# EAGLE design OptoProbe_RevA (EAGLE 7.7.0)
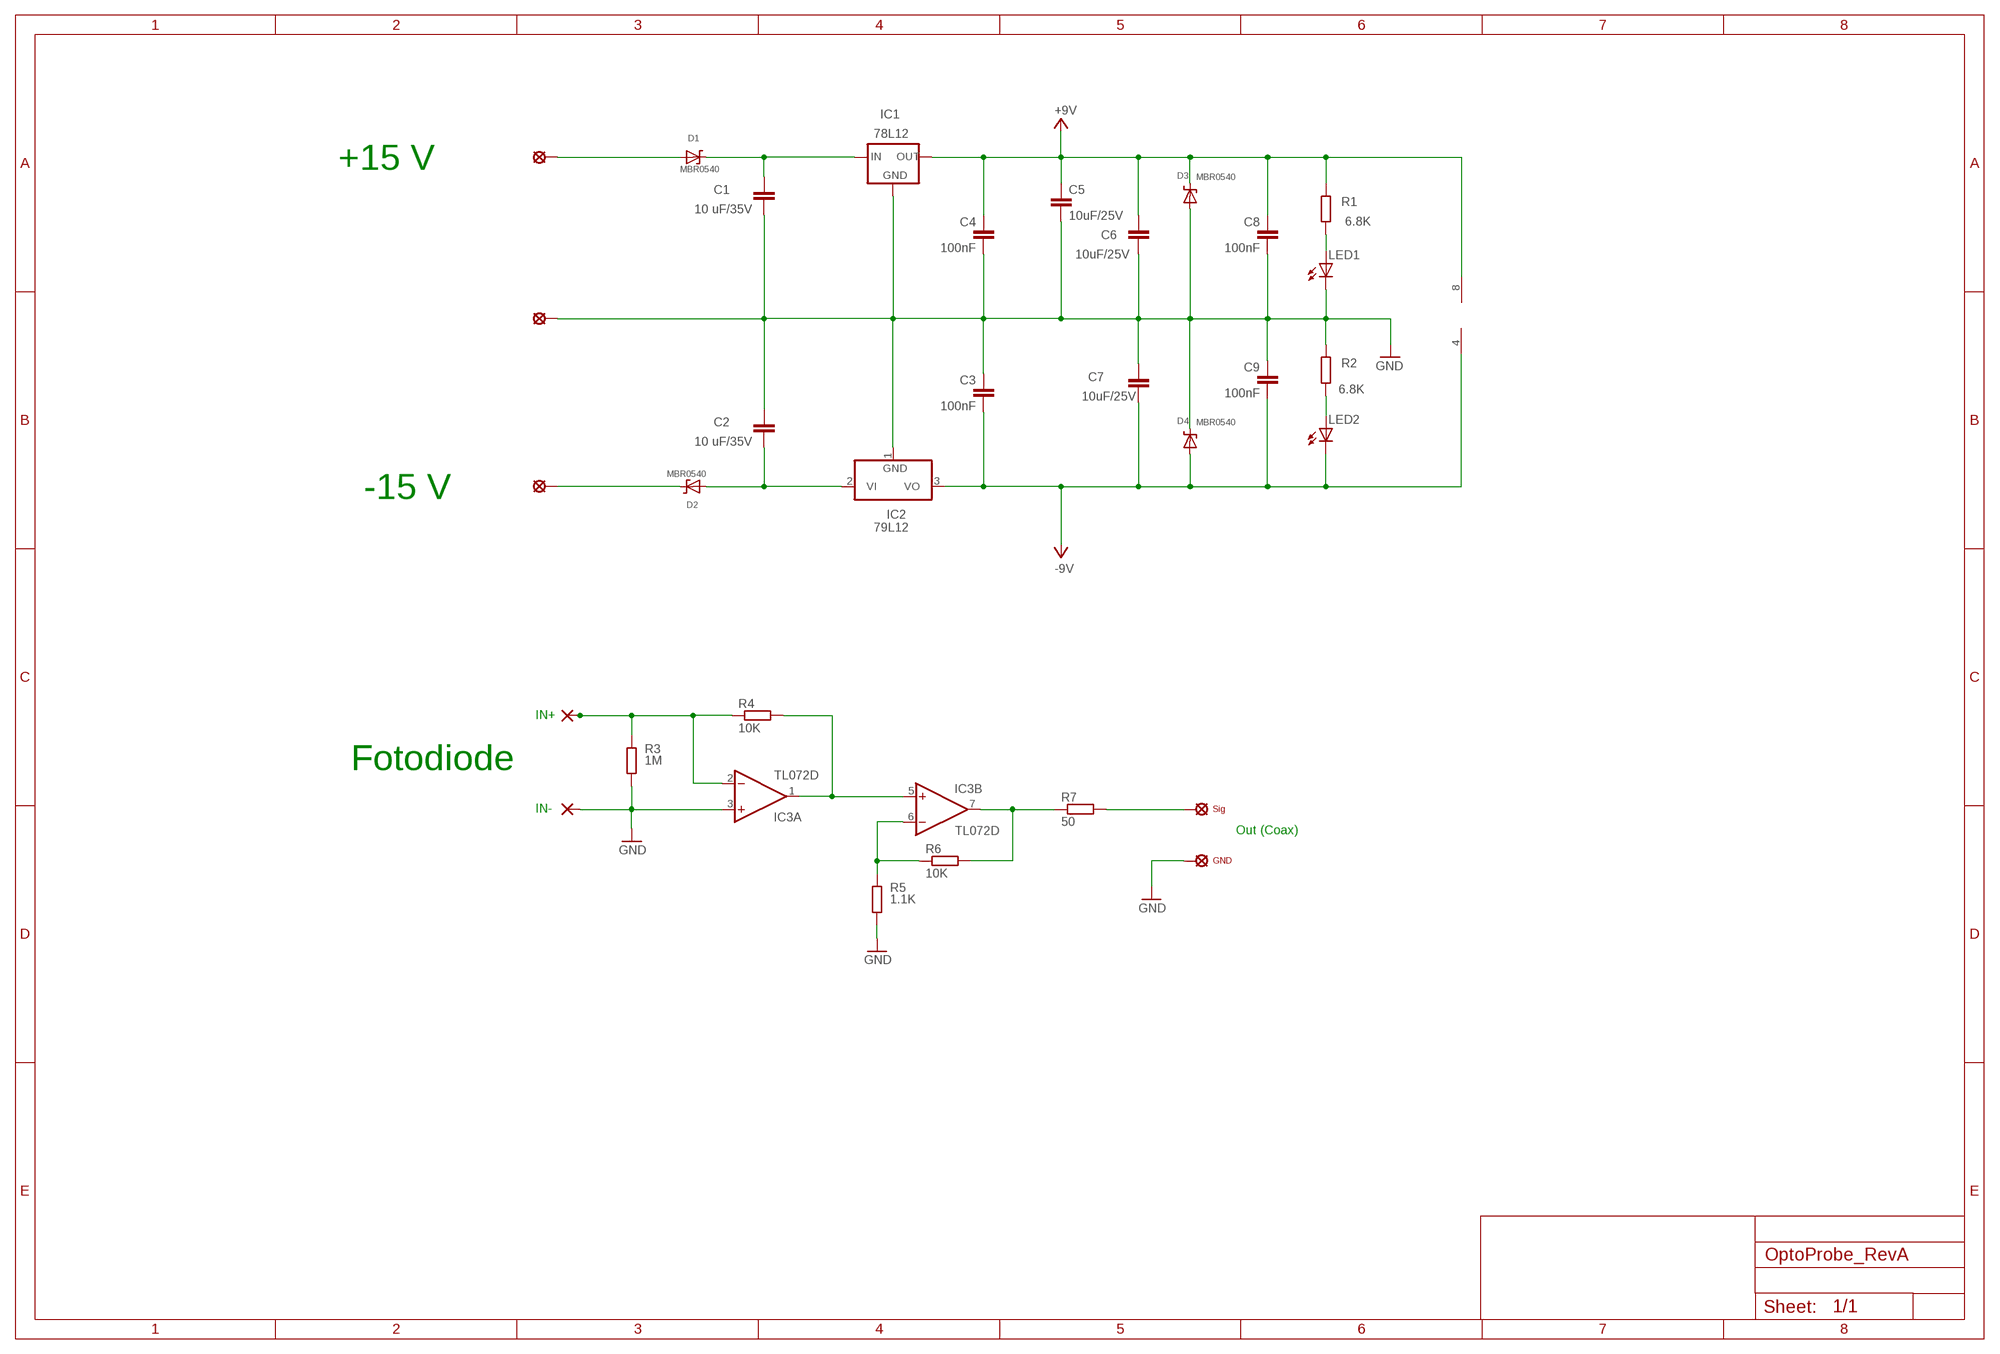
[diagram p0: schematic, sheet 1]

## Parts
+5VIN  SE2.5_1.0  [SE2.5_1.0]
C1  10 uF/35V  C-EUC1206  [C1206]
C2  10 uF/35V  C-EUC1206  [C1206]
C3  100nF  C-EUC0603  [C0603]
C4  100nF  C-EUC0603  [C0603]
C5  10uF/25V  C-EUC0805  [C0805]
C6  10uF/25V  C-EUC0805  [C0805]
C7  10uF/25V  C-EUC0805  [C0805]
C8  100nF  C-EUC0603  [C0603]
C9  100nF  C-EUC0603  [C0603]
D1  MBR0540  D-SCHTTKY_PMEG2005EH_SOD-123  [SOD-123]
D2  MBR0540  D-SCHTTKY_PMEG2005EH_SOD-123  [SOD-123]
D3  MBR0540  D-SCHTTKY_PMEG2005EH_SOD-123  [SOD-123]
D4  MBR0540  D-SCHTTKY_PMEG2005EH_SOD-123  [SOD-123]
GND  SE2.5_1.0  [SE2.5_1.0]
GND3  SE2.5_1.0  [SE2.5_1.0]
IC1  78L12  78LXX  [78LXX]
IC2  79L12  79L05Z  [TO92]
IC3  TL072D  [SO08]
IN+  SMD3X2  [SMD3.00X2.00]
IN-  SMD3X2  [SMD3.00X2.00]
LED1  LEDCHIPLED_0603  [CHIPLED_0603]
LED2  LEDCHIPLED_0603  [CHIPLED_0603]
R1  6.8K  R-EU_R0603  [R0603]
R2  6.8K  R-EU_R0603  [R0603]
R3  1M  R-EU_R0603  [R0603]
R4  10K  R-EU_R0603  [R0603]
R5  1.1K  R-EU_R0603  [R0603]
R6  10K  R-EU_R0603  [R0603]
R7  50  R-EU_R0603  [R0603]
U$3  RG178BU  [RG178BU]

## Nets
+9V: C4.1 C5.1 C6.1 C8.1 D3.K IC1.OUT IC3.8(P:V+) R1.1
+11.5V: C1.1 D1.K IC1.IN
-9V: C3.2 C7.2 C9.2 D4.A IC2.3(VO) IC3.4(P:V-) LED2.C
GND: C1.2 C2.1 C3.1 C4.2 C5.2 C6.2 C7.1 C8.2 C9.1 D3.A D4.K GND.MP IC1.GND IC2.1(GND) IC3.3(A:+IN) IN-.1(P) LED1.C R2.1 R3.2 R5.2 U$3.P$3(GND) U$3.P$4(GND) U$3.P$5(GND) U$3.P$6(GND) U$3.P$7(GND) U$3.P$8(GND) U$3.P$9(GND) U$3.P$10(GND)
N$1: C2.2 D2.A IC2.2(VI)
N$2: LED2.A R2.2
N$3: D2.K GND3.MP
N$5: IC3.2(A:-IN) IN+.1(P) R3.1 R4.1
N$6: IC3.1(A:OUT) IC3.5(B:+IN) R4.2
N$7: IC3.6(B:-IN) R5.1 R6.1
N$8: IC3.7(B:OUT) R6.2 R7.1
N$16: LED1.A R1.2
N$29: +5VIN.MP D1.A
N$34: R7.2 U$3.P$1(SIG) U$3.P$2(SIG)

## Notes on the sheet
- +15 V
- -15 V
- Fotodiode
- Out (Coax)

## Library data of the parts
+5VIN GND GND3 = solpad2:SE2.5_1.0: SOLDER PAD
C1-C9 = rcl:C-EU: CAPACITOR, European symbol
D1-D4 = diodes:D-SCHTTKY_*_: Schottky diode; LOAD: 500mA; PARTNO: DIS-PMEG2005EH; RATE: 355mW; SIZE: (SOD-123); VAL: PMEG2005EH; VOLT: 20V
IC1 = v-reg:78LXX: VOLTAGE REGULATOR
IC2 = linear:79*: Negative VOLTAGE REGULATOR
IC3 = linear:TL072: OP AMP
IN+ IN- = wirepad2:SMD3X2: SMD PAD 3x2mm
LED1 LED2 = led2:LED: LED
R1-R7 = rcl:R-EU_: RESISTOR, European symbol
U$3 = solpad2:RG178BU: SMD-Pads für SMA-Koaxkabel RG178BU

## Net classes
3 gnd: clearance 0.12 mm to class 0, clearance 0.3 mm to class 1, clearance 0.1 mm to class 2

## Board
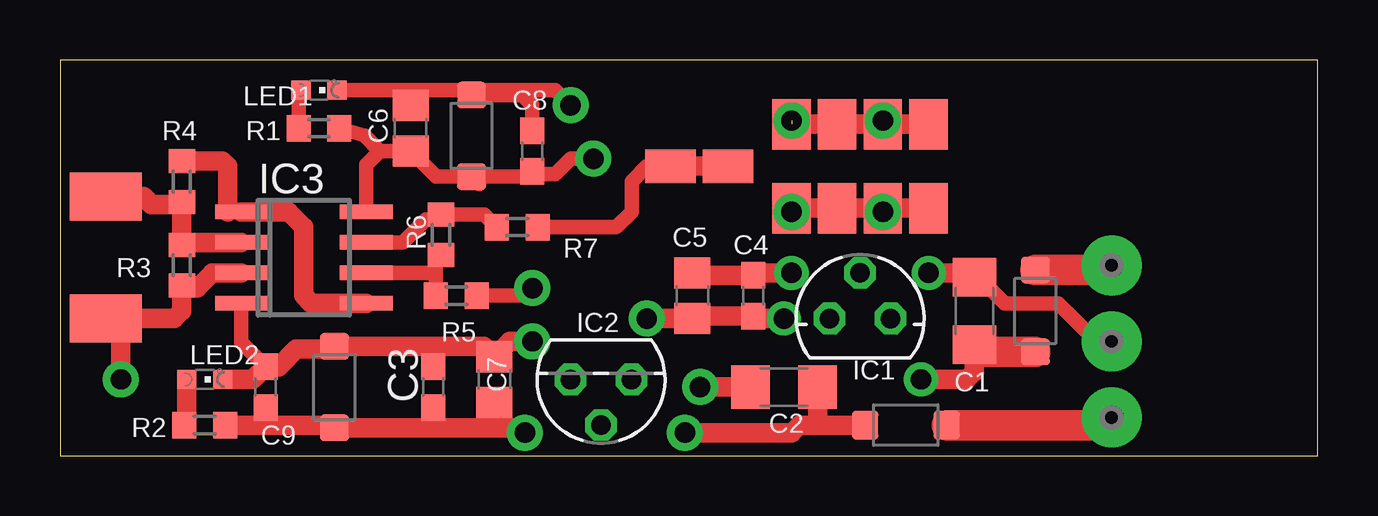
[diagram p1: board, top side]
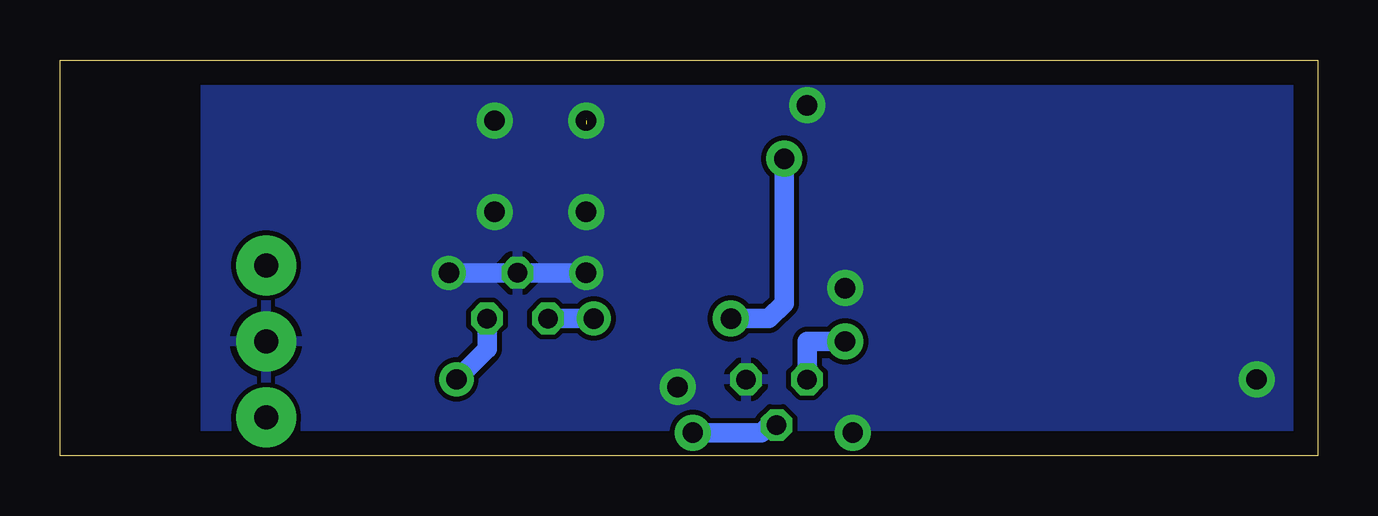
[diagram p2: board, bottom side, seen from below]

Size 52.4 x 16.5 mm. Coordinates in mm from the lower left corner, seen from the top.
Outline: 0,0 52.4,0 52.4,16.5 0,16.5 0,0
Copper layers (1*16): Top 0.035mm / dielectric 1.5mm / Bottom 0.035mm
Design rules "default": minimum track width 10mil, minimum drill 24mil, track to track 8mil, track to pad 8mil, pad to pad 8mil, via to via 8mil, smd to smd 8mil, copper to edge 40mil, drill to drill 8mil, minimum pad ring 10mil, minimum via ring 8mil, stop-mask expansion 4mil, vias tented up to drill 0mil, thermal gap 10mil

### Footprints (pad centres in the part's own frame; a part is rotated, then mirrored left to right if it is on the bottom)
SE2.5_1.0 = drill 1 pad 2.5: MP 0,0
C1206 = smd 1.6 x 1.8: 1 -1.4,0; 2 1.4,0
C0603 = smd 1.1 x 1: 1 -0.85,0; 2 0.85,0
C0805 = smd 1.3 x 1.5: 1 -0.95,0; 2 0.95,0
SOD-123 = smd 1.1 x 1.2: A 1.7,0; K -1.7,0
78LXX = drill 0.813 octagon: GND 0,1.905; IN 1.27,0; OUT -1.27,0
TO92 = drill 0.813 octagon: 1 -1.27,0; 2 0,1.905; 3 1.27,0
SO08 = smd 0.6 x 2.2: 1 -1.905,-2.6; 2 -0.635,-2.6; 3 0.635,-2.6; 4 1.905,-2.6; 5 1.905,2.6; 6 0.635,2.6; 7 -0.635,2.6; 8 -1.905,2.6
SMD3.00X2.00 = smd 2 x 3: 1 0,0
CHIPLED_0603 = smd 0.8 x 0.8: A 0,-0.75; C 0,0.75
R0603 = smd 1 x 1.1: 1 -0.85,0; 2 0.85,0
RG178BU = smd 1.4 x 2.1: P$1 0,6; P$2 0,3.6 | smd 2.1 x 1.6: P$3 -1.75,0.95; P$4 1.75,0.95; P$5 -1.75,-0.95; P$6 1.75,-0.95; P$7 -1.75,-2.85; P$8 1.75,-2.85; P$9 -1.75,-4.75; P$10 1.75,-4.75

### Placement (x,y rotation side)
+5VIN  43.81,7.94 0 top
C1  38.1,6.03 90 top
C2  30.16,2.86 0 top
C3  15.56,2.86 90 top
C4  28.89,6.67 90 top
C5  26.35,6.67 90 top
C6  14.61,13.65 90 top
C7  18.1,3.17 90 top
C8  19.69,12.7 90 top
C9  8.57,2.86 90 top
D1  40.64,6.03 90 top
D2  35.24,1.27 180 top
D3  17.14,13.34 90 top
D4  11.43,2.86 90 top
GND  43.81,4.76 0 top
GND3  43.81,1.59 0 top
IC1  33.34,5.71 0 top
IC2  22.54,3.17 180 top
IC3  10.16,8.26 270 top
IN+  1.91,10.79 90 top
IN-  1.91,5.71 90 top
LED1  10.8,15.24 270 top
LED2  6.03,3.17 270 top
R1  10.8,13.65 180 top
R2  6.03,1.27 180 top
R3  5.08,7.94 270 top
R4  5.08,11.43 90 top
R5  16.51,6.67 0 top
R6  15.88,9.21 90 top
R7  19.05,9.53 0 top
U$3  31.43,12.06 90 top

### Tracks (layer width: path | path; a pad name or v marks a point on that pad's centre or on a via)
+9V  (via drill 0.85 pad 1.42, 0.85 pad 1.5)
  Top 0.61: 17.46,11.32 D3.K | D3.K 19.47,11.63 C8.1 19.79,11.75 20.64,11.75 21.27,12.38 v22.22,12.38 | D3.K 15.67,11.63 C6.1 13.33,12.7 | 13.33,12.7 12.7,13.34 R1.1 | IC3.8 12.76,12.13 13.33,12.7
  Top 0.813: v24.45,5.71 v24.45,5.72 C5.1 26.45,5.82 C4.1 29,5.71 v30.16,5.71
  Bottom 0.813: v24.45,5.71 22.86,5.71 22.22,6.35 v22.22,12.38 | IC1.OUT v30.16,5.71
+11.5V  (via drill 0.85 pad 1.42)
  Top 0.813: v35.88,3.17 37.78,3.17 38.1,3.49 C1.1
  Top 1.27: D1.K 38.4,4.33 C1.1
  Bottom 0.813: IC1.IN 34.61,4.45 v35.88,3.17
-9V  (via drill 0.85 pad 1.5)
  Top 0.406: 14.27,4.56 14.23,4.6 | 17.67,4.56 C7.2
  Top 0.61: IC3.4 7.56,4.72 C9.2
  Top 0.813: D4.A 14.27,4.56 | D4.A 15.56,4.56 | 15.56,4.56 17.67,4.56 | LED2.C 8.04,3.17 C9.2 9.11,3.71 9.84,4.45 11.32,4.45 D4.A | v19.69,4.76 18.74,4.76 C7.2 | C3.2 15.56,4.56
  Bottom 0.813: IC2.3 21.27,4.76 v19.69,4.76
GND  (via drill 0.85 pad 1.42, 0.85 pad 1.5)  (1 unrouted)
  Top 0.406: 5.71,6.99 5.18,6.99 R3.2
  Top 0.61: 14.61,15.24 LED1.C 20.64,15.24 v21.27,14.61 | 14.61,15.24 16.94,15.24 D3.A 19.26,15.04 19.69,14.61 C8.2 | C6.2 14.61,15.24 | C1.2 38.29,7.43 39.37,6.35 41.59,6.35 43.18,4.76 GND.MP | R5.2 19.37,6.67 v19.69,6.99
  Top 0.813: U$3.P$4 U$3.P$6 U$3.P$8 U$3.P$10 | U$3.P$3 U$3.P$5 U$3.P$7 U$3.P$9 | C5.2 26.45,7.52 C4.2 29,7.62 v30.48,7.62 | C2.1 v26.67,2.86 | C1.2 38.1,7.62 v36.19,7.62 | IC3.3 6.35,7.62 5.71,6.99 | IN-.1 2.54,5.71 | R3.2 5.08,6.03 4.76,5.71 2.54,5.71 | R2.1 8.57,1.27 | 8.57,1.27 11.32,1.27 D4.K 15.56,1.16 | C9.1 8.57,1.27 | 15.56,1.16 18.1,1.16 | 18.1,1.16 19.16,1.16 v19.37,0.95 | C7.1 18.1,1.16 | C3.1 15.56,1.16 | 2.54,5.71 v2.54,3.17
  Top 1.27: U$3.P$7 v34.28,10.17 v34.29,10.16
  Bottom 0.813: v30.48,7.62 IC1.GND v36.19,7.62
  other vias: 30.48,10.16 34.29,13.97 30.48,13.97
  pour Bottom: 0.32,0 0.32,16.51 46.36,16.51 46.36,0
N$1  (via drill 0.85 pad 1.5)
  Top 0.813: D2.A 31.75,1.27 | 31.75,1.27 30.8,1.27 30.48,0.95 v26.03,0.95 | C2.2 31.56,1.46 31.75,1.27
  Bottom 0.813: IC2.2 22.86,1.27 23.18,0.95 v26.03,0.95
N$2
  Top 0.813: LED2.A 5.28,1.37 R2.2
N$3
  Top 1.27: D2.K 43.5,1.27 GND3.MP
N$5
  Top 0.406: 4.98,10.48 R4.1
  Top 0.813: IC3.2 5.18,8.89 R3.1 R4.1 | IN+.1 3.49,10.79 3.81,10.48 4.98,10.48
N$6
  Top 0.406: 6.99,10.16 IC3.1
  Top 0.813: R4.2 6.77,12.28 6.99,12.06 6.99,10.16 | IC3.1 9.52,10.16 10.16,9.53 10.16,6.67 10.48,6.35 IC3.5
N$7
  Top 0.61: R5.1 15.66,7.62 | 15.66,7.62 15.66,8.14 R6.1 | IC3.6 15.66,7.62
N$8
  Top 0.61: IC3.7 14.29,8.89 15.24,9.84 15.66,9.84 R6.2 17.67,10.06 R7.1
N$16
  Top 0.61: R1.2 9.94,15.14 LED1.A
N$29
  Top 1.27: D1.A 43.61,7.73 +5VIN.MP
N$34
  Top 0.61: R7.2 23.18,9.53 23.81,10.16 23.81,11.43 24.45,12.06 U$3.P$1
  Top 0.813: U$3.P$1 U$3.P$2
